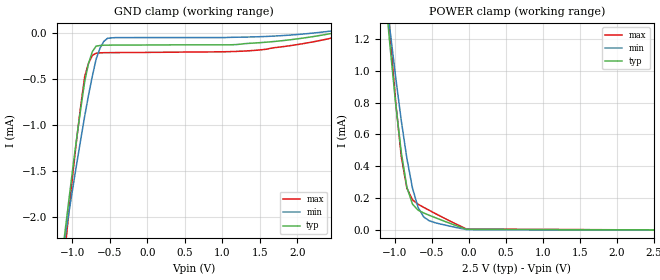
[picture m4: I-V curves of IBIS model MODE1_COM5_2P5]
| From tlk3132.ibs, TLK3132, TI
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[Model]   MODE1_COM5_2P5
Model_type   Input
Polarity   Non-Inverting
Vinl =  0.7V
Vinh =  1.7V
C_comp   0.5589689p   0.5151173p   0.6105178p
[Model Spec]
Vinl   0.7V   0.7V   0.7V
Vinh   1.7V   1.7V   1.7V
[Temperature Range]   25   105   0
[Voltage Range]   2.5   2.25   2.75
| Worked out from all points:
|   GND clamp passes 1 mA (typ) near -0.92 V on its own axis
|   POWER clamp passes 1 mA (typ) near -1.03 V on its own axis
[POWER_clamp]
|   voltage   I(typ)   I(min)   I(max)
-2.5V     9.469mA    7.499mA    11.6mA
-1.086V   1.284mA    1.359mA    1.398mA
-1.061V   1.154mA    1.256mA    1.238mA
-984.8mV  795.8uA    961uA      807.2uA
-909.1mV  488.5uA    688.4uA    462.3uA
-833.3mV  268.9uA    450.4uA    262.4uA
-757.6mV  162.6uA    263uA      189.7uA
-681.8mV  124.4uA    141.6uA    161.9uA
-606.1mV  106.6uA    81.82uA    142uA
-530.3mV  92.08uA    57.64uA    123.2uA
-25.25mV  4.064uA    2.273uA    5.631uA
2.5V      20.47nA    14.17nA    153.6nA
[GND_clamp]
|   voltage   I(typ)   I(min)   I(max)
-2.5V     -11.97mA   -9.829mA   -13.99mA
-1.136V   -2.439mA   -2.439mA   -2.697mA
-1.086V   -2.096mA   -2.173mA   -2.285mA
-1.035V   -1.758mA   -1.911mA   -1.881mA
-934.3mV  -1.109mA   -1.396mA   -1.113mA
-833.3mV  -529.3uA   -904.2uA   -474.4uA
-782.8mV  -334.1uA   -679.6uA   -330.7uA
-681.8mV  -145.4uA   -286.3uA   -222.7uA
-580.8mV  -135.3uA   -95.42uA   -217uA
-530.3mV  -134.7uA   -60.56uA   -216.4uA
1.338V    -116.2uA   -46.62uA   -196.9uA
2.449V    -7.76uA    18.68uA    -58.92uA
